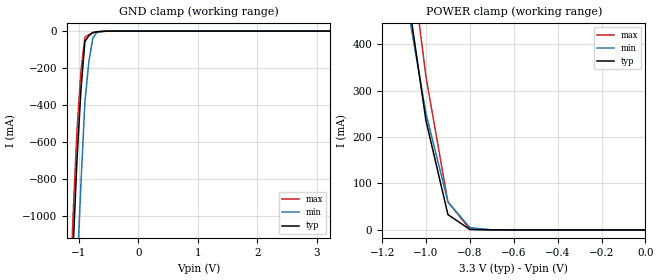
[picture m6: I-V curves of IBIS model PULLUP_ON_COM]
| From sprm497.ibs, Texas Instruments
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|   Model Cell PULLUP_ON_COM
[Model]   PULLUP_ON_COM
Model_type   Input
Polarity   Non-Inverting
Vinl =  0.8
Vinh =  2
C_comp   0.8695239p   0.8563616p   0.8781626p
[Model Spec]
Vinl   0.8   0.8   0.8
Vinh   2   2   2
[Temperature Range]   25   105   0
[Voltage Range]   3.3   3.14   3.47
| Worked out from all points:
|   GND clamp passes 1 mA (typ) near -0.58 V on its own axis
|   POWER clamp passes 1 mA (typ) near -0.79 V on its own axis
[POWER_clamp]
|   voltage   I(typ)   I(min)   I(max)
-3.3V     9.572A     8.243A     10.54A
-1.067V   452.2mA    433.3mA    579.4mA
-1.033V   343.6mA    341.7mA    454.3mA
-1V       234.9mA    250.2mA    329.2mA
-900mV    33.09mA    60.44mA    60.09mA
-800mV    1.079mA    4.959mA    1.736mA
-700mV    81.06uA    300.6uA    96.17uA
-11.55fV  364pA      4.312nA    654.5pA
[GND_clamp]
|   voltage   I(typ)   I(min)   I(max)
-3.3V     -22.43A    -23.04A    -22.26A
-1.167V   -1.763A    -2.446A    -1.569A
-1.1V     -1.191A    -1.863A    -1.003A
-1.033V   -696.7mA   -1.322A    -538.1mA
-966.7mV  -318.5mA   -829.3mA   -215.1mA
-900mV    -56.21mA   -384.9mA   -33.6mA
-833.3mV  -25.22mA   -165.5mA   -18.63mA
-766.7mV  -7.763mA   -39.46mA   -9.039mA
-700mV    -3.851mA   -6.791mA   -4.843mA
-633.3mV  -2.011mA   -3.394mA   -2.522mA
3.233V    -4.892uA   4.971uA    -20.1uA
